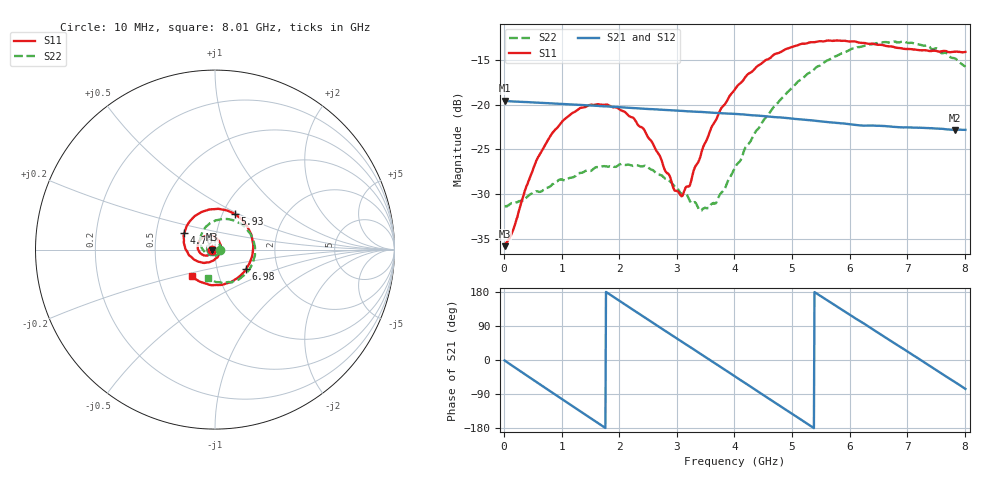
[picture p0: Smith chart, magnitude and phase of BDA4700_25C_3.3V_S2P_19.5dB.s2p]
!Agilent Technologies,E5071B,MY42404982,A.09.10
!Date: Mon Oct 20 18:11:14 2025
!Data & Calibration Information:
!Freq	S11:SOLT2(ON)	S21:SOLT2(ON)	S12:SOLT2(ON)	S22:SOLT2(ON)
# Hz S RI R 50
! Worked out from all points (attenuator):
!   801 points, 10 MHz to 8.01 GHz, reference 50 ohm
!   highest |S21| = -19.58 dB at 10 MHz (marker M1); lowest = -22.8 dB at 7.83 GHz (marker M2)
!   lowest |S11| = -35.8 dB at 10 MHz (marker M3), VSWR 1.03, Z = 48.4 - j0.108 ohm
!   |S11| at or under -10 dB: start of sweep to end of sweep
!   |S22| runs from -31.9 to -13.0 dB; largest |S21 - S12| = 0.0013
!   S11 on the Smith chart (normalised r, x): 10 MHz: 0.97, -0.00; 4.76 GHz: 0.70, +0.13; 5.93 GHz: 1.14, +0.48; 6.98 GHz: 1.38, -0.31; 8.01 GHz: 0.74, -0.23
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1e7  -0.0162 -0.00111  0.1049 -0.0023  0.1048 -0.00234  0.0271 -0.000866
1.5e8  -0.0173 -0.00952  0.1001 -0.0283  0.1001 -0.0283  0.0271 -0.00741
7e8  -0.0482 -0.0333  0.0314 -0.0971  0.0314 -0.097  0.00569 -0.0333
1.03e9  -0.0783 -0.0233  -0.0271 -0.097  -0.027 -0.097  -0.0174 -0.0336
1.35e9  -0.0961 0.0057  -0.0739 -0.0665  -0.0739 -0.0666  -0.0378 -0.0173
2.08e9  -0.0511 0.076  -0.0822 0.0502  -0.0822 0.0503  -0.0286 0.0361
2.42e9  -0.00633 0.0731  -0.0394 0.0862  -0.0394 0.0863  -0.00202 0.0452
2.68e9  0.0211 0.0488  0.00216 0.0938  0.00202 0.0937  0.0163 0.0374
2.96e9  0.0317 0.00958  0.0449 0.0808  0.0449 0.0807  0.0284 0.0204
3.1e9  0.0288 -0.0114  0.063 0.0671  0.0625 0.0675  0.0304 0.00844
3.4e9  0.0032 -0.05  0.0868 0.0271  0.087 0.0271  0.0215 -0.0138
3.54e9  -0.0168 -0.0638  0.0903 0.00537  0.0903 0.00524  0.0127 -0.0232
3.69e9  -0.0433 -0.0712  0.088 -0.0178  0.088 -0.0181  -0.000808 -0.0285
4.01e9  -0.1052 -0.0612  0.0645 -0.0609  0.0646 -0.0607  -0.0349 -0.0275
4.76e9  -0.1712 0.0909  -0.04 -0.0748  -0.0397 -0.075  -0.0814 0.0627
5.35e9  -0.0655 0.2128  -0.0814 -0.00462  -0.0814 -0.00512  -0.0141 0.1524
5.93e9  0.109 0.1986  -0.0461 0.063  -0.0464 0.0628  0.1209 0.1551
6.68e9  0.2107 -0.0131  0.0446 0.0608  0.0448 0.0609  0.2221 -0.00687
6.98e9  0.1744 -0.1063  0.0677 0.0314  0.0677 0.0309  0.2043 -0.0876
7.44e9  0.0482 -0.1936  0.0691 -0.0258  0.0691 -0.0257  0.108 -0.1723
7.83e9  -0.0796 -0.1808  0.0379 -0.0614  0.0379 -0.0616  0.00522 -0.1807
8.01e9  -0.1288 -0.1486  0.0172 -0.0701  0.0174 -0.0702  -0.0375 -0.1579
